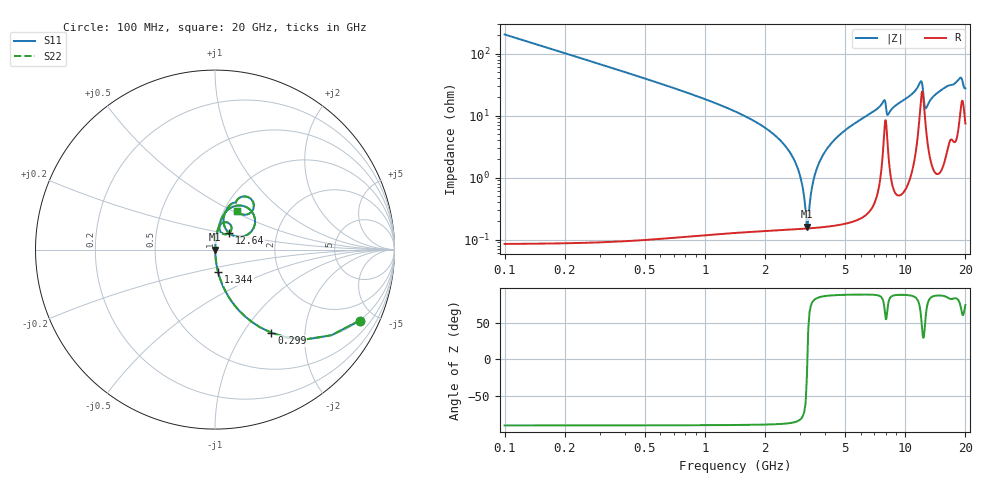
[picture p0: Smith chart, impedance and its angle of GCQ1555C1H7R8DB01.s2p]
!Murata Part Number: GCQ1555C1H7R8DB01
!These Parameters are Measured in Series Mode Connection
!Data Generated on Jan 08, 2026
!  o--ll--o
!Port1  Port2
!  o------o
!Operation Temp=25[degC], DC Bias Voltage=0[V]
!Freq. Start=100[MHz] Stop=20[GHz] 401[Steps]
# Hz S RI R 50
!Freq.(Hz) S11(Real) S11(Imag) S21(Real) S21(Imag) S12(Real) S12(Imag) S22(Real) S22(Imag)
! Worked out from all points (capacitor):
!   401 points, 100 MHz to 20 GHz, reference 50 ohm
!   read as one part in series: C = 7.8 pF near 199.5 MHz
!   lowest |Z| = 162 mohm at 3.234 GHz (marker M1)
!   series resonance near 3.249 GHz, so ESL is about 310 pH
!   S11 on the Smith chart (normalised r, x): 100 MHz: 1.00, -4.08; 299 MHz: 1.00, -1.35; 1.344 GHz: 1.00, -0.25; 12.64 GHz: 1.15, +0.21; 20 GHz: 1.15, +0.53
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1e8  0.8059 -0.3953  0.1941 0.3953  0.1941 0.3953  0.8059 -0.3953
2.99e8  0.3142 -0.4635  0.6858 0.4635  0.6858 0.4635  0.3142 -0.4635
5.975e8  0.0989 -0.2969  0.9011 0.2969  0.9011 0.2969  0.0989 -0.2969
1.34375e9  0.0168 -0.1236  0.9832 0.1236  0.9832 0.1236  0.0168 -0.1236
2.687e9  0.00202 -0.0241  0.998 0.0241  0.998 0.0241  0.00202 -0.0241
2.9855e9  0.00159 -0.0107  0.9984 0.0107  0.9984 0.0107  0.00159 -0.0107
3.23425e9  0.0015 -0.000587  0.9985 0.000587  0.9985 0.000587  0.0015 -0.000587
3.33375e9  0.00152 0.00324  0.9985 -0.00324  0.9985 -0.00324  0.00152 0.00324
3.43325e9  0.00157 0.00697  0.9984 -0.00697  0.9984 -0.00697  0.00157 0.00697
3.73175e9  0.00187 0.0176  0.9981 -0.0176  0.9981 -0.0176  0.00187 0.0176
4.32875e9  0.00303 0.0371  0.997 -0.0371  0.997 -0.0371  0.00303 0.0371
6.7665e9  0.0149 0.108  0.9851 -0.108  0.9851 -0.108  0.0149 0.108
7.81125e9  0.0609 0.1526  0.9391 -0.1526  0.9391 -0.1526  0.0609 0.1526
8.20925e9  0.0369 0.0929  0.9631 -0.0929  0.9631 -0.0929  0.0369 0.0929
1.005e10  0.0394 0.1779  0.9606 -0.1779  0.9606 -0.1779  0.0394 0.1779
1.19405e10  0.1928 0.2246  0.8072 -0.2246  0.8072 -0.2246  0.1928 0.2246
1.23385e10  0.1659 0.0755  0.8341 -0.0755  0.8341 -0.0755  0.1659 0.0755
1.2637e10  0.0789 0.0917  0.9211 -0.0917  0.9211 -0.0917  0.0789 0.0917
1.338325e10  0.0478 0.1662  0.9522 -0.1662  0.9522 -0.1662  0.0478 0.1662
1.67165e10  0.1142 0.2613  0.8858 -0.2613  0.8858 -0.2613  0.1142 0.2613
1.885575e10  0.1989 0.2832  0.8011 -0.2832  0.8011 -0.2832  0.1989 0.2832
2e10  0.1224 0.2158  0.8776 -0.2158  0.8776 -0.2158  0.1224 0.2158
